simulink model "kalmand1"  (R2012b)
settings: Solver=ode45  StartTime=0.0  StopTime=100  RelTol=1e-3
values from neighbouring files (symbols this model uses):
  dt = 0.01    [aktiv_tilger_1.m]    (also in aktiv_tilger_12.m; aktiv_tilger_2.m; beobachter_1.m; beobachter_2.m)
  dtn = 0.01    [kalman_1.m]    (also in kalman_10.m; kalman_11.m; kalman_12.m; kalman_d1.m)
  Kest = kalman(P,1,0.01),    [LQG_1.m]    (also in ss_zwei_eing_1.m = kalman(sys2, Q, R))
  ki = -Kn(n+1)    [beobachter_2.m]    (also in beobachter_22.m; kalman_12.m = -Kn(3); kalman_13.m = -Kn(4); kalman_d1.m = -Kn(4))
  Kr = 2000    [aktiv_tilger_2.m]    (also in beobachter_22.m = 5; fuellstnd_3.m = 10,; fuellstnd_31.m = 10,; kalman_12.m = Kn(1:2))
  sys2 = sys1(:,[1,1,1])    [kalman_11.m]    (also in kalman_12.m; kalman_13.m = sys1(:,[1,1,1,1]); kalman_2.m = ss(H2); kalman_3.m = ss(H2))
  Ts = 0.001    [fuellstnd_3.m]    (also in fuellstnd_31.m; kalman_d1.m = 0.05; kalman_d2.m = 0.1; kalman_d3.m = 0.1)
  vnd = 1e-4    (= 0.0001)    [kalman_1.m]    (also in kalman_10.m; kalman_11.m; kalman_12.m; kalman_13.m = 0.01)
  vny = 1e-6    (= 1e-06)    [kalman_1.m]    (also in kalman_10.m; kalman_11.m = ', num2str(vny),' )']); kalman_12.m = ', num2str(vny),' )']); kalman_13.m = ', num2str(vny),' )']))
  x0 = [30,-20,0,0,0,0]    [beobachter_1.m]    (also in beobachter_2.m = [0,0,0,0,0.3,0]; beobachter_22.m = [0.1,0,0.1,0,0.3,0]; kalman_13.m = zeros(1,3); kalman_d1.m = zeros(1,3))
undefined symbols (not defined in the file or in its folder): DiscIntNeverNeededParam
libraries: simulink x2, dspstat3 x1

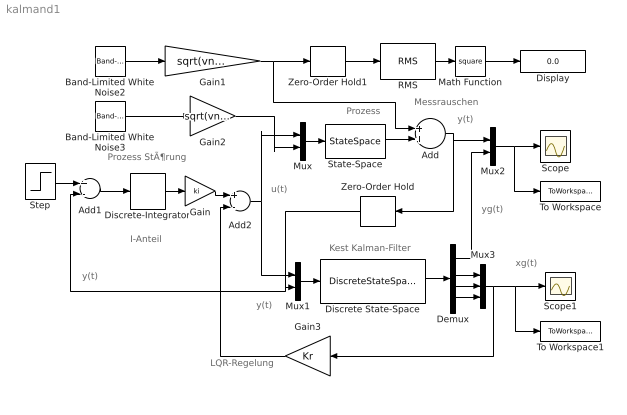
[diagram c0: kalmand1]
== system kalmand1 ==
  note: I-Anteil
  note: LQR-Regelung
  note: y(t)
  note: y(t)
  note: xg(t)
  note: u(t)
  note: y(t)
  note: yg(t)
  note: Messrauschen
  note: Prozess StÃ¶rung
  note: Kest Kalman-Filter
  note: Prozess
  Add : Sum
  Add1 : Sum  Inputs=+-
  Add2 : Sum  Inputs=+-
  Band-Limited White Noise2 : simulink/Sources/Band-Limited White Noise  Cov=dtn  Ts=dtn  seed=[23341]
  Band-Limited White Noise3 : simulink/Sources/Band-Limited White Noise  Cov=[dtn, dtn, dtn]  Ts=dtn  seed=[23341, 2785, 3672]
  Demux : Demux
  Discrete State-Space : DiscreteStateSpace  A=Kest.a  B=Kest.b  C=Kest.c  D=Kest.d  SampleTime=Ts
  Discrete-Integrator : DiscreteIntegrator  SampleTime=Ts  ICPrevOutput=DiscIntNeverNeededParam  ICPrevScaledInput=DiscIntNeverNeededParam
  Display : Display
  Gain : Gain  Gain=ki
  Gain1 : Gain  Gain=sqrt(vny/dtn)
  Gain2 : Gain  Gain=sqrt(vnd/dtn)*eye(3,3)  Multiplication=Matrix(K*u)
  Gain3 : Gain  Gain=Kr  Multiplication=Matrix(K*u)
  Math Function : Math  Operator=square
  Mux : Mux  Inputs=2
  Mux1 : Mux  Inputs=2
  Mux2 : Mux  Inputs=2
  Mux3 : Mux  Inputs=3
  RMS : dspstat3/RMS  run=on  reset_popup=None  InputProcessing=Columns as channels (frame based)  directionMode=Each column  dimension=1  treatSBRowAsCol=on
  Scope : Scope
  Scope1 : Scope
  State-Space : StateSpace  A=sys2.a  B=sys2.b  C=sys2.c  D=sys2.d  X0=x0
  Step : Step  After=step  SampleTime=Ts
  To Workspace : ToWorkspace  VariableName=y  SampleTime=-1  SaveFormat=Structure With Time
  To Workspace1 : ToWorkspace  VariableName=y1  SampleTime=-1  SaveFormat=Structure With Time
  Zero-Order Hold : ZeroOrderHold  SampleTime=Ts
  Zero-Order Hold1 : ZeroOrderHold  SampleTime=dt
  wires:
  Mux/1 -> State-Space/1
  Gain2/1 -> Mux/2
  State-Space/1 -> Add/2
  Mux1/1 -> Discrete State-Space/1
  Discrete State-Space/1 -> Demux/1
  Mux2/1 -> To Workspace/1, Scope/1
  Demux/1 -> Mux2/2
  Demux/3 -> Mux3/2
  Mux3/1 -> Gain3/1, To Workspace1/1, Scope1/1
  Step/1 -> Add1/1
  Discrete-Integrator/1 -> Gain/1
  Gain/1 -> Add2/1
  Add2/1 -> Mux1/1, Mux/1
  Demux/4 -> Mux3/3
  Zero-Order Hold/1 -> Add1/2, Mux1/2
  Add/1 -> Zero-Order Hold/1, Mux2/1
  Add1/1 -> Discrete-Integrator/1
  Band-Limited White Noise3/1 -> Gain2/1
  Gain1/1 -> Zero-Order Hold1/1, Add/1
  RMS/1 -> Math Function/1
  Math Function/1 -> Display/1
  Zero-Order Hold1/1 -> RMS/1
  Band-Limited White Noise2/1 -> Gain1/1
  Demux/2 -> Mux3/1
  Gain3/1 -> Add2/2
